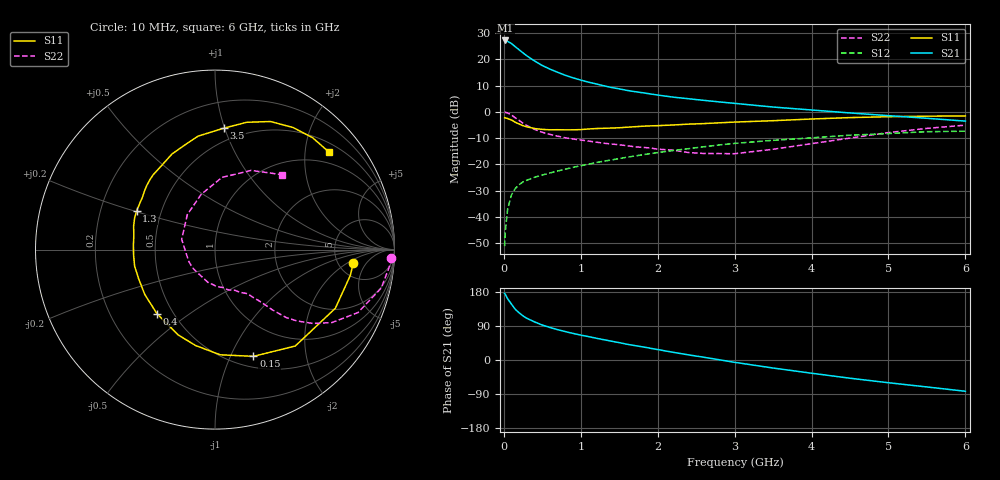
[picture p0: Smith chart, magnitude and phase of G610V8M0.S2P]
! SIEMENS Small Signal Semiconductors
! BFG193
! Si NPN RF Bipolar Junction Transistor in SOT223
! VCE = 10 V  IC = 8 mA
! Common Emitter S-Parameters:  August  1996
# GHz  S  MA  R  50
!  f  S11  S21  S12  S22
! GHz  MAG  ANG  MAG  ANG  MAG  ANG  MAG  ANG
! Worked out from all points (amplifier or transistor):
!   36 points, 10 MHz to 6 GHz, reference 50 ohm
!   highest |S21| = 27.1 dB at 20 MHz (marker M1)
!   |S21| within 3 dB of that: start of sweep to 175.5 MHz
!   unconditionally stable (mu >= 1): 976.8 MHz to 2.538 GHz
!   at 250 MHz: K = 0.46, MSG = 24.5 dB, |S12| = -26.6 dB
!   at 1.4 GHz: K = 1.07, MAG = 12.2 dB, |S12| = -18.3 dB
!   at 6 GHz: K = 0.85, MSG = 1.9 dB, |S12| = -7.4 dB
!   S11 on the Smith chart (normalised r, x): 10 MHz: 6.93, -2.52; 150 MHz: 0.62, -1.22; 400 MHz: 0.41, -0.38; 1.3 GHz: 0.36, +0.20; 3.5 GHz: 0.40, +1.00; 6 GHz: 0.71, +2.55
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0.01  0.7744 -5.4  22.73 175.7  0.0028 93.5  0.984 -2.6
0.02  0.7676 -10.8  22.74 173.0  0.0055 85.8  0.9774 -5.3
0.05  0.7459 -26.0  21.86 161.4  0.0144 77.3  0.9509 -13.0
0.1  0.699 -50.2  19.84 147.2  0.0265 68.5  0.87 -23.8
0.15  0.6322 -70.2  17.23 133.5  0.0351 59.1  0.7674 -32.0
0.2  0.5867 -87.2  15.08 124.3  0.0415 55.1  0.6839 -37.0
0.25  0.5451 -101.5  13.17 116.2  0.0467 51.4  0.6061 -41.0
0.3  0.5178 -113.3  11.58 109.9  0.0503 49.7  0.5503 -43.6
0.4  0.4817 -132.2  9.248 100.5  0.0571 47.7  0.4638 -46.4
0.5  0.4644 -147.3  7.588 92.2  0.0629 46.6  0.409 -48.0
0.6  0.4557 -158.7  6.485 85.8  0.069 47.2  0.3724 -49.5
0.7  0.4572 -168.4  5.634 80.0  0.075 47.7  0.3448 -51.2
0.9  0.4553 176.5  4.431 70.1  0.0882 47.4  0.3042 -53.8
1.1  0.472 163.9  3.668 61.7  0.101 47.0  0.2782 -59.1
1.3  0.4868 153.7  3.13 53.5  0.1155 46.1  0.2531 -63.8
1.6  0.5105 140.3  2.558 41.6  0.1372 43.0  0.2274 -74.5
2.2  0.5628 119.7  1.904 20.4  0.1841 34.7  0.1867 -102.2
2.8  0.6184 103.0  1.545 0.6  0.2348 23.9  0.1611 -142.2
3.5  0.6789 85.7  1.233 -21.2  0.2875 8.6  0.1945 162.7
4.5  0.7776 66.6  0.953 -48.1  0.36 -11.2  0.3176 104.0
5.5  0.8273 48.9  0.754 -71.1  0.4193 -35.9  0.4854 65.4
6  0.836 40.4  0.667 -82.5  0.4285 -50.4  0.5585 48.4
